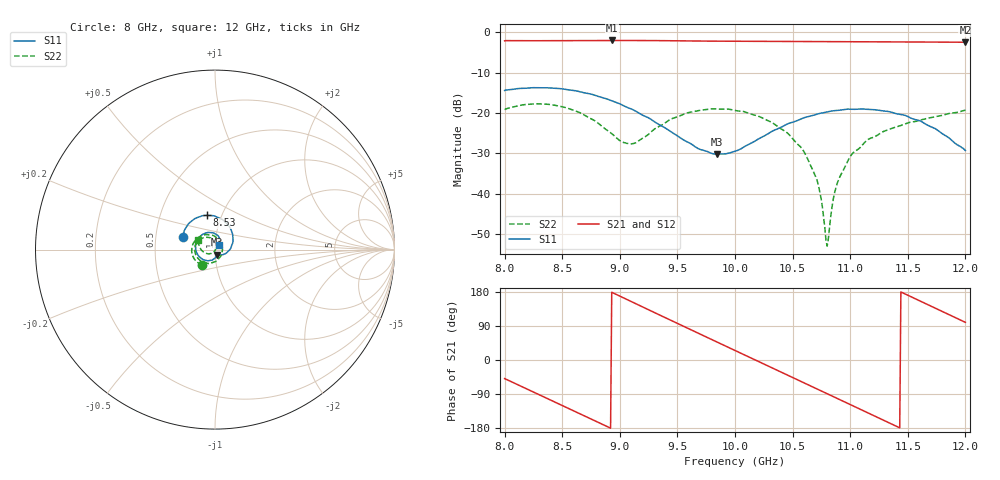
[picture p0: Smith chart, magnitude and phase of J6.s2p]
!Keysight Technologies,N5234A,MY52241180,A.10.60.03
!Date: Tuesday, May 30, 2023 15:23:55
!Correction: S11(Full 2 Port(1,2))
!S21(Full 2 Port(1,2))
!S12(Full 2 Port(1,2))
!S22(Full 2 Port(1,2))
!S2P File: Measurements: S11, S21, S12, S22:
# Hz S  dB  R 50
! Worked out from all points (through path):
!   401 points, 8 GHz to 12 GHz, reference 50 ohm
!   highest |S21| = -2.01 dB at 8.93 GHz (marker M1); lowest = -2.5 dB at 12 GHz (marker M2)
!   group delay of S21, straight-line fit = 397 ps
!   lowest |S11| = -30.2 dB at 9.84 GHz (marker M3), VSWR 1.06, Z = 51.3 - j2.87 ohm
!   |S11| at or under -10 dB: start of sweep to end of sweep
!   |S22| runs from -53.0 to -17.7 dB; largest |S21 - S12| = 0.0015
!   S11 on the Smith chart (normalised r, x): 8 GHz: 0.69, +0.10; 8.53 GHz: 0.85, +0.34; 12 GHz: 1.04, +0.06
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8e9  -14.41 158.5  -2.11 -49.1  -2.11 -49.1  -19.17 -129.9
8.27e9  -13.72 133.2  -2.08 -87.2  -2.09 -87.2  -17.71 -171.7
8.53e9  -14.15 103.7  -2.06 -124.0  -2.07 -124.0  -18.65 146.9
8.67e9  -14.84 86.2  -2.04 -144.0  -2.05 -144.0  -20.14 121.9
8.93e9  -16.97 50.9  -2.01 178.7  -2.03 178.7  -25.09 59.9
9.11e9  -19.11 24.9  -2.02 152.8  -2.03 152.7  -27.60 -13.5
9.34e9  -22.84 -9.0  -2.06 119.6  -2.07 119.5  -23.35 -91.2
9.58e9  -27.08 -43.1  -2.13 85.1  -2.13 85.1  -20.03 -137.6
9.84e9  -30.18 -64.8  -2.20 48.0  -2.21 48.0  -19.00 -177.7
1e10  -29.50 -74.5  -2.23 25.2  -2.24 25.2  -19.36 159.6
1.032e10  -24.56 -103.6  -2.27 -20.3  -2.28 -20.3  -22.30 117.4
1.057e10  -21.49 -137.4  -2.29 -56.0  -2.30 -56.0  -28.40 84.5
1.067e10  -20.64 -151.2  -2.30 -70.3  -2.31 -70.3  -33.82 69.5
1.073e10  -20.12 -160.1  -2.30 -78.9  -2.31 -78.9  -38.74 56.7
1.078e10  -19.86 -167.3  -2.31 -86.0  -2.32 -86.1  -48.52 29.0
1.08e10  -19.73 -169.6  -2.31 -88.9  -2.32 -88.9  -52.99 -24.9
1.088e10  -19.37 178.3  -2.32 -100.3  -2.33 -100.4  -38.11 -115.1
1.099e10  -19.03 163.4  -2.33 -116.1  -2.34 -116.1  -31.27 -131.9
1.115e10  -19.08 140.0  -2.35 -139.0  -2.36 -139.0  -26.66 -149.5
1.134e10  -19.67 113.6  -2.37 -166.2  -2.38 -166.2  -24.03 -165.1
1.164e10  -22.48 74.1  -2.41 150.9  -2.41 150.9  -21.51 173.2
1.2e10  -29.29 53.5  -2.45 99.3  -2.46 99.3  -19.30 150.9
